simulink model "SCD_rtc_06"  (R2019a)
settings: configuration reference "configurationSettings" (kept in a data dictionary, not in this file)
undefined symbols (not defined in the file or in its folder): algo_demo1_fp, SCDnode06params, signal1, signal2

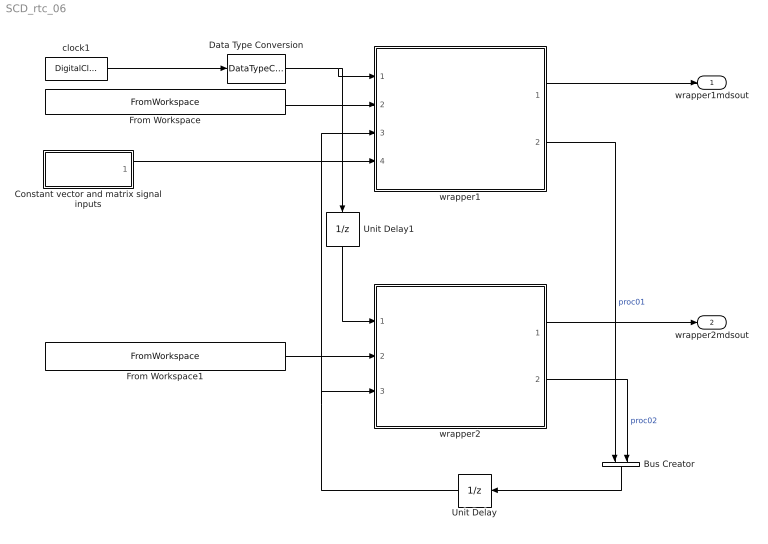
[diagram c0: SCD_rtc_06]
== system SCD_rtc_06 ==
  Bus Creator : BusCreator  Inputs=2
  Constant vector and matrix signal inputs : Subsystem
  Data Type Conversion : DataTypeConversion  OutDataTypeStr=single
  From Workspace : FromWorkspace  VariableName=SCDsimdata.SCDnode0601_simdata.wavegen  OutDataTypeStr=Bus: WG0601bus  SampleTime=SCDnode06params.timing.dt  Interpolate=off  OutputAfterFinalValue=Holding final value
  From Workspace1 : FromWorkspace  VariableName=SCDsimdata.SCDnode0602_simdata.wavegen  OutDataTypeStr=Bus: WG0602bus  SampleTime=SCDnode06params.timing.dt  Interpolate=off  OutputAfterFinalValue=Holding final value
  Unit Delay : UnitDelay  SampleTime=-1  HasFrameUpgradeWarning=on
  Unit Delay1 : UnitDelay  SampleTime=-1  HasFrameUpgradeWarning=on
  clock1 : DigitalClock  SampleTime=algo_demo1_fp.timing.dt
  wrapper1 : ModelReference  ModelNameDialog=SCDwrap_demo1.slx  SimulationMode=Normal  ModelReferenceVersion=1.33
  wrapper2 : ModelReference  ModelNameDialog=SCDwrap_demo2.slx  SimulationMode=Normal  ModelReferenceVersion=1.14
  wrapper1mdsout : Outport  OutDataTypeStr=Bus: mdsout01
  wrapper2mdsout : Outport  Port=2  OutDataTypeStr=Bus: mdsout02
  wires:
  wrapper1/1 -> wrapper1mdsout/1
  wrapper2/1 -> wrapper2mdsout/1
  wrapper1/2 -> Bus Creator/1  "proc01"
  wrapper2/2 -> Bus Creator/2  "proc02"
  Bus Creator/1 -> Unit Delay/1
  Unit Delay/1 -> wrapper2/3, wrapper1/3
  From Workspace/1 -> wrapper1/2
  clock1/1 -> Data Type Conversion/1
  Data Type Conversion/1 -> wrapper1/1, Unit Delay1/1
  From Workspace1/1 -> wrapper2/2
  Unit Delay1/1 -> wrapper2/1
  Constant vector and matrix signal inputs/1(Out1) -> wrapper1/4

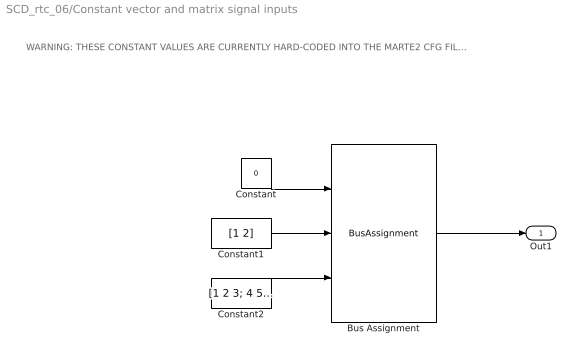
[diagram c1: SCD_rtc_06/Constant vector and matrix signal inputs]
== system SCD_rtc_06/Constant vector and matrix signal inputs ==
  note: WARNING: THESE CONSTANT VALUES ARE CURRENTLY HARD-CODED INTO THE MARTE2 CFG FILE SOURCE: rtapp-thread1.cfgsrc CHANGES MUST BE REFLECTED THERE TO HAVE CONSISTENT SIMULATION-REALTIME RUN EQUIVALENCE
  Bus Assignment : BusAssignment  AssignedSignals=signal1,signal2
  Constant : Constant  Value=0  OutDataTypeStr=Bus: vecmatin
  Constant1 : Constant  Value=[1 2]  OutDataTypeStr=single
  Constant2 : Constant  Value=[1 2 3; 4 5 6]  OutDataTypeStr=single
  Out1 : Outport
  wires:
  Constant2/1 -> Bus Assignment/3
  Constant1/1 -> Bus Assignment/2
  Constant/1 -> Bus Assignment/1
  Bus Assignment/1 -> Out1/1
